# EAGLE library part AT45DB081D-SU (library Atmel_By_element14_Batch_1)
8-megabit DataFlash
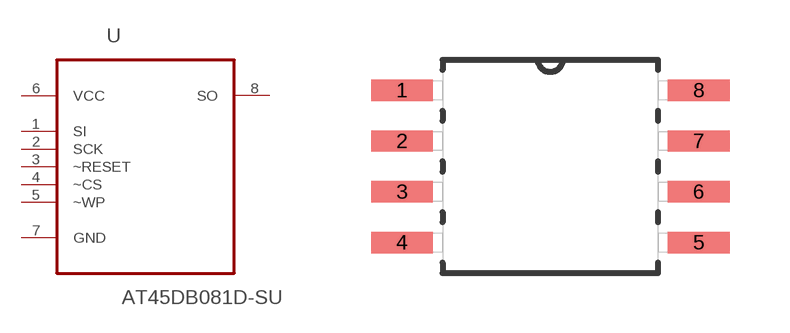
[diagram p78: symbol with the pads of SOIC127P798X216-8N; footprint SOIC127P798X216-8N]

Designator prefix U

## AT45DB081D-SU (MPN: AT45DB081D-SU; OC_FARNELL: 1455039; OC_NEWARK: 58M3837; PACKAGE: SOIC-8; SUPPLIER: Atmel)  [SOIC127P798X216-8N]
1  SI  in
2  SCK  in
3  ~RESET  in
4  ~CS  in
5  ~WP  in
6  VCC  pwr
7  GND  pas
8  SO  out

## Footprint SOIC127P798X216-8N (pad centres in mm)
smd 1.549 x 0.533: 1 -3.708,1.905; 2 -3.708,0.635; 3 -3.708,-0.635; 4 -3.708,-1.905; 5 3.708,-1.905; 6 3.708,-0.635; 7 3.708,0.635; 8 3.708,1.905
